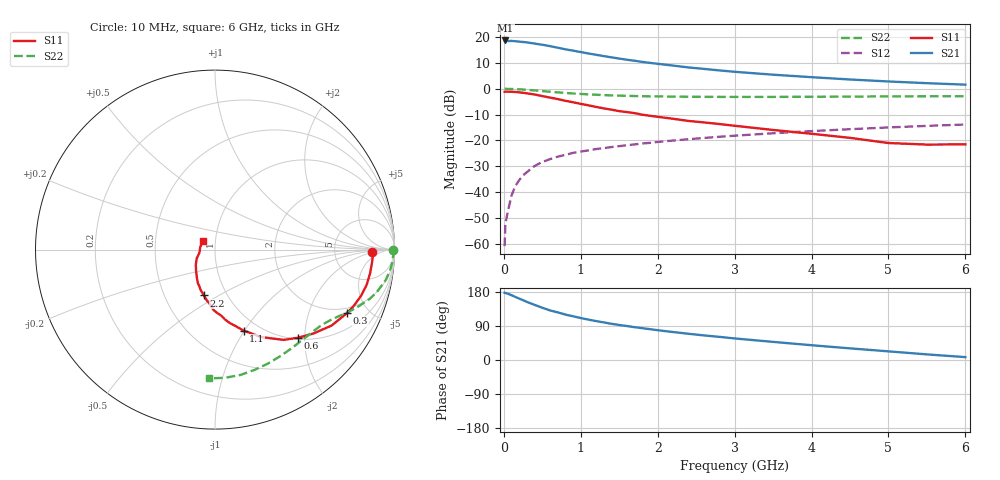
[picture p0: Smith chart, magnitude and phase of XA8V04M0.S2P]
! SIEMENS Discrete & RF Semiconductors
! BFY180
! Si NPN RF Bipolar Junction Transistor in MICRO-X
! VCE = 8 V  IC = 4 mA
! Common Emitter S-Parameters:  May  1997
# GHz  S  MA  R  50
!  f  S11  S21  S12  S22
! GHz  MAG  ANG  MAG  ANG  MAG  ANG  MAG  ANG
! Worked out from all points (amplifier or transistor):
!   36 points, 10 MHz to 6 GHz, reference 50 ohm
!   highest |S21| = 18.7 dB at 20 MHz (marker M1)
!   |S21| within 3 dB of that: start of sweep to 731.9 MHz
!   unconditionally stable (mu >= 1): 2.314 GHz to end of sweep
!   at 250 MHz: K = 0.18, MSG = 25.8 dB, |S12| = -33.5 dB
!   at 1.4 GHz: K = 0.81, MSG = 17.4 dB, |S12| = -22.6 dB
!   at 6 GHz: K = 1.05, MAG = 6.3 dB, |S12| = -13.8 dB
!   S11 on the Smith chart (normalised r, x): 10 MHz: 15, -2; 300 MHz: 1.72, -3.64; 600 MHz: 1.03, -1.86; 1.1 GHz: 0.85, -0.99; 2.2 GHz: 0.78, -0.43; 6 GHz: 0.87, +0.09
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0.01  0.8759 -0.8  8.562 177.4  0.0009 81.2  0.9931 -0.2
0.02  0.8807 -1.7  8.614 176.8  0.0024 82.9  0.9999 -0.8
0.05  0.8785 -4.2  8.39 175.1  0.0041 83.9  0.9933 -2.0
0.1  0.874 -8.8  8.432 171.0  0.0086 86.3  0.9896 -4.1
0.15  0.8673 -13.2  8.317 166.4  0.0132 83.4  0.9844 -6.1
0.3  0.8166 -25.6  7.914 153.3  0.0244 75.8  0.9536 -11.7
0.4  0.7753 -33.1  7.493 145.5  0.0321 71.5  0.9309 -14.9
0.5  0.7216 -40.3  7.123 137.9  0.0383 67.3  0.9042 -17.7
0.6  0.6754 -46.6  6.688 130.9  0.0435 64.9  0.876 -20.1
0.8  0.585 -57.7  5.806 119.9  0.0526 59.8  0.8309 -24.1
1  0.5095 -66.5  5.137 110.7  0.061 56.6  0.7947 -27.3
1.1  0.4786 -70.6  4.819 106.6  0.0642 55.5  0.7794 -28.6
1.3  0.4179 -78.5  4.281 99.2  0.0711 53.5  0.7546 -31.3
1.5  0.3696 -84.6  3.846 92.4  0.0776 51.8  0.7366 -33.9
1.8  0.3147 -94.1  3.313 84.0  0.0874 50.3  0.7191 -37.6
2.2  0.2631 -103.6  2.81 73.8  0.0996 47.5  0.7061 -42.6
2.4  0.2387 -109.6  2.589 69.2  0.1056 46.2  0.7008 -45.1
2.8  0.208 -117.5  2.268 61.1  0.1179 43.9  0.6966 -49.9
3.5  0.1597 -131.3  1.874 47.8  0.1378 39.0  0.6963 -58.7
4.5  0.1123 -154.7  1.513 30.7  0.1652 32.0  0.7053 -71.7
5.5  0.0832 169.4  1.284 14.8  0.1914 24.3  0.7165 -85.6
6  0.0841 143.2  1.202 7.6  0.2034 20.1  0.7181 -92.6
